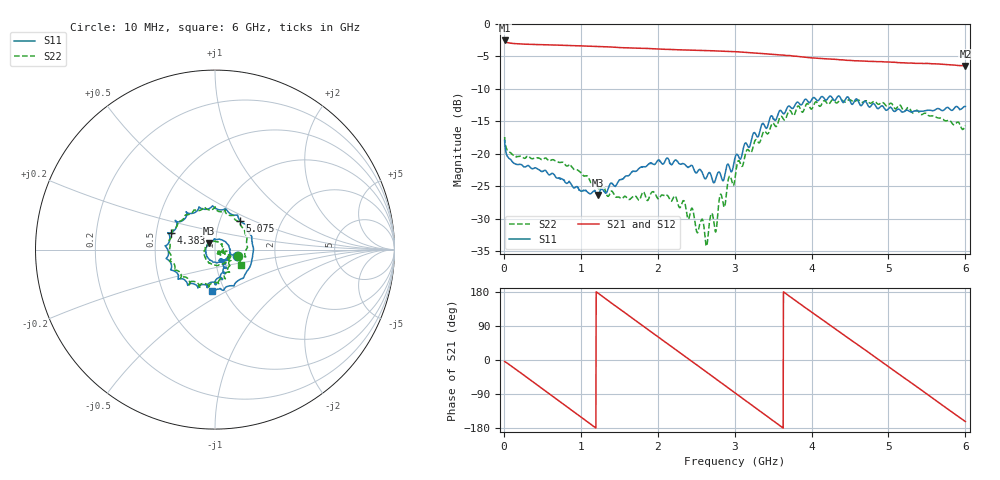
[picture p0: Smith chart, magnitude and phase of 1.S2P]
!Agilent Technologies,E5071C,MY46316741,A.11.02
!Date: Tue Oct 20 14:43:48 2020
!Data & Calibration Information:
!Freq	S11:SOLT4(ON)	S21:SOLT4(ON)	S12:SOLT4(ON)	S22:SOLT4(ON)
!PortZ  Port1:50+j0  Port2:50+j0
!Above PortZ is port z conversion or system Z0 setting when saving the data.
!When reading, reference impedance value at option line is always used.
# Hz S dB R 50
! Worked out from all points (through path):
!   1561 points, 10 MHz to 6 GHz, reference 50 ohm
!   highest |S21| = -2.53 dB at 10 MHz (marker M1); lowest = -6.5 dB at 6 GHz (marker M2)
!   group delay of S21, straight-line fit = 408 ps
!   lowest |S11| = -26.3 dB at 1.22 GHz (marker M3), VSWR 1.10, Z = 46.6 + j3.21 ohm
!   |S11| at or under -10 dB: start of sweep to end of sweep
!   |S22| runs from -34.2 to -11.6 dB; largest |S21 - S12| = 0.0052
!   S11 on the Smith chart (normalised r, x): 10 MHz: 1.27, -0.10; 4.383 GHz: 0.59, +0.12; 5.075 GHz: 1.25, +0.42; 6 GHz: 0.87, -0.43
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1e7  -17.90 -17.5  -2.53 -4.2  -2.58 -4.1  -17.41 -15.0
2.595833e8  -22.00 -41.7  -3.09 -39.9  -3.13 -39.9  -20.65 -33.0
5.360449e8  -22.52 -81.6  -3.19 -81.1  -3.23 -81.1  -20.62 -66.7
7.625897e8  -23.91 -120.0  -3.27 -114.8  -3.30 -114.9  -21.27 -98.5
1.012173e9  -25.75 -173.1  -3.37 -152.0  -3.39 -152.1  -23.07 -138.8
1.219519e9  -26.31 134.7  -3.46 177.1  -3.48 177.0  -25.13 -179.3
1.645731e9  -23.05 41.8  -3.68 114.1  -3.69 113.9  -26.91 75.6
2.006667e9  -20.94 -13.3  -3.86 60.7  -3.87 60.6  -26.91 -0.5
2.248571e9  -21.05 -41.9  -3.95 25.1  -3.97 24.9  -27.06 -32.0
2.482795e9  -22.77 -58.4  -4.04 -9.3  -4.07 -9.6  -30.34 -40.8
2.636385e9  -23.62 -69.4  -4.09 -32.0  -4.12 -32.3  -34.16 -37.3
2.693981e9  -23.30 -58.4  -4.12 -40.5  -4.15 -40.9  -29.26 -24.1
3.005e9  -20.60 -59.4  -4.26 -87.0  -4.30 -87.2  -23.78 -26.5
3.239224e9  -16.96 -68.7  -4.45 -121.8  -4.48 -121.9  -18.92 -46.4
3.527205e9  -14.84 -93.1  -4.69 -164.4  -4.72 -164.6  -15.70 -72.9
4.007173e9  -11.54 -154.2  -5.21 125.6  -5.22 125.4  -13.03 -136.4
4.383468e9  -11.54 159.4  -5.51 71.3  -5.54 71.1  -11.63 -178.8
4.709846e9  -12.03 110.1  -5.72 24.6  -5.75 24.4  -11.80 143.2
5.001667e9  -13.00 59.2  -5.83 -17.8  -5.87 -17.8  -12.45 106.3
5.074622e9  -13.45 48.7  -5.88 -28.3  -5.93 -28.3  -12.89 100.3
5.520032e9  -13.27 -26.5  -6.07 -92.7  -6.09 -92.7  -14.09 43.8
6e9  -12.70 -93.6  -6.45 -162.5  -6.45 -162.4  -15.64 -30.5
